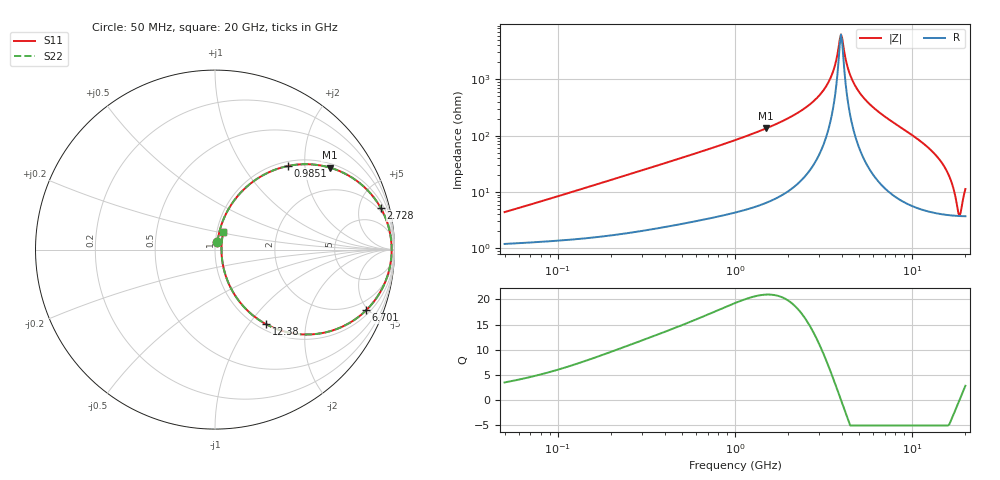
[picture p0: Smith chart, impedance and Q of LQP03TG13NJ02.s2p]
!Murata Part Number: LQP03TG13NJ02
!These Parameters are Measured in Series Mode Connection
!  o--[Z]--o
!Port1  Port2
!  o-------o
!Freq. Start=50[MHz] Stop=20[GHz], 401[Steps]
# Hz S RI R 50
!Freq.(Hz) S11(Real) S11(Imag) S21(Real) S21(Imag) S12(Real) S12(Imag) S22(Real) S22(Imag)
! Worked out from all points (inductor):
!   401 points, 50 MHz to 20 GHz, reference 50 ohm
!   read as one part in series: L = 13.4 nH near 51.52 MHz
!   highest Q = 21 at 1.498 GHz (marker M1), where L = 14.3 nH
!   self-resonance near 3.967 GHz
!   S11 on the Smith chart (normalised r, x): 50 MHz: 1.02, +0.08; 985.1 MHz: 1.09, +1.64; 2.728 GHz: 1.56, +7.77; 6.701 GHz: 1.27, -4.86; 12.38 GHz: 1.09, -1.21; 20 GHz: 1.07, +0.21
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5e7  0.0136 0.0413  0.9864 -0.0413  0.9864 -0.0413  0.0136 0.0413
1.364002e8  0.0266 0.1079  0.9734 -0.1079  0.9734 -0.1079  0.0266 0.1079
3.721004e8  0.1003 0.2648  0.8997 -0.2648  0.8997 -0.2648  0.1003 0.2648
9.85133e8  0.4065 0.4658  0.5935 -0.4658  0.5935 -0.4658  0.4065 0.4658
1e9  0.4141 0.4673  0.5859 -0.4673  0.5859 -0.4673  0.4141 0.4673
1.498439e9  0.6388 0.4571  0.3612 -0.4571  0.3612 -0.4571  0.6388 0.4571
2.728004e9  0.9236 0.2322  0.0764 -0.2322  0.0764 -0.2322  0.9236 0.2322
3.415248e9  0.9741 0.098  0.0259 -0.098  0.0259 -0.098  0.9741 0.098
3.626126e9  0.9806 0.0597  0.0194 -0.0597  0.0194 -0.0597  0.9806 0.0597
3.967106e9  0.9843 0.00082  0.0157 -0.00082  0.0157 -0.00082  0.9843 0.00082
4.087748e9  0.9839 -0.0191  0.0161 0.0191  0.0161 0.0191  0.9839 -0.0191
4.405649e9  0.9792 -0.0691  0.0208 0.0691  0.0208 0.0691  0.9792 -0.0691
4.748272e9  0.969 -0.1194  0.031 0.1194  0.031 0.1194  0.969 -0.1194
6.701223e9  0.842 -0.338  0.158 0.338  0.158 0.338  0.842 -0.338
7.442007e9  0.7745 -0.3929  0.2255 0.3929  0.2255 0.3929  0.7745 -0.3929
9.745021e9  0.5383 -0.4723  0.4617 0.4723  0.4617 0.4723  0.5383 -0.4723
1.238412e10  0.2839 -0.4152  0.7161 0.4152  0.7161 0.4152  0.2839 -0.4152
1.573793e10  0.0826 -0.2029  0.9174 0.2029  0.9174 0.2029  0.0826 -0.2029
1.696185e10  0.05 -0.1119  0.95 0.1119  0.95 0.1119  0.05 -0.1119
1.828096e10  0.0365 -0.0162  0.9635 0.0162  0.9635 0.0162  0.0365 -0.0162
1.88369e10  0.0366 0.0223  0.9634 -0.0223  0.9634 -0.0223  0.0366 0.0223
2e10  0.0459 0.0981  0.9541 -0.0981  0.9541 -0.0981  0.0459 0.0981
